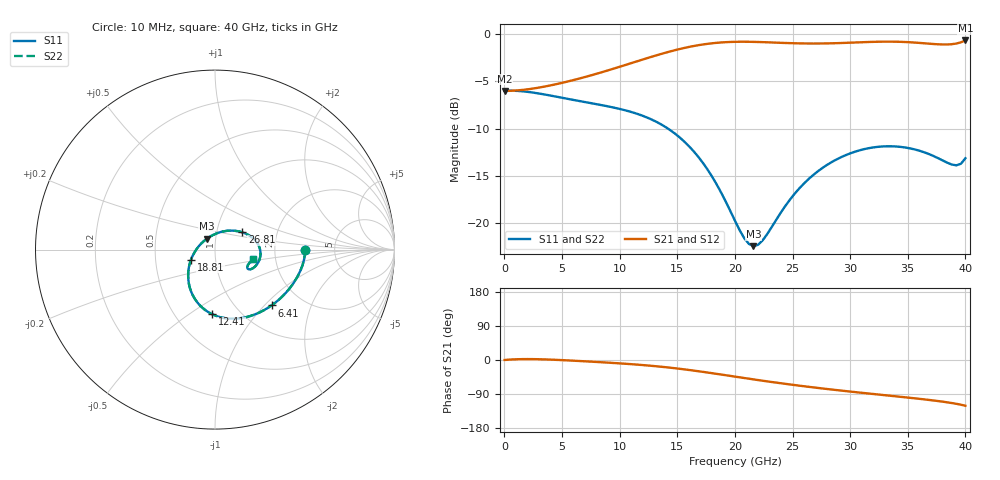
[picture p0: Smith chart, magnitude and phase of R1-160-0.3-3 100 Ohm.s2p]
!version-1
!date-09.2020
# MHz S RI R 50
!Freq ReS11 ImS11 ReS21 ImS21 ReS12 ImS12 ReS22 ImS22
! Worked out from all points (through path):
!   101 points, 10 MHz to 40 GHz, reference 50 ohm
!   highest |S21| = -0.70 dB at 40 GHz (marker M1); lowest = -6.0 dB at 10 MHz (marker M2)
!   group delay of S21, straight-line fit = 9.25 ps
!   lowest |S11| = -22.4 dB at 21.61 GHz (marker M3), VSWR 1.16, Z = 45.3 + j5.51 ohm
!   |S11| at or under -10 dB: 14.18 GHz to end of sweep
!   |S22| runs from -22.4 to -6.0 dB; largest |S21 - S12| = 0
!   S11 on the Smith chart (normalised r, x): 10 MHz: 3.00, -0.00; 6.41 GHz: 1.42, -1.10; 12.41 GHz: 0.75, -0.62; 18.81 GHz: 0.76, -0.09; 26.81 GHz: 1.33, +0.26; 40 GHz: 1.53, -0.18
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10  0.5 -0.000398  0.5 0.000242  0.5 0.000242  0.5 -0.000398
2810  0.466 -0.1382  0.5176 0.0194  0.5176 0.0194  0.466 -0.1382
6410  0.3153 -0.3111  0.5782 -0.0255  0.5782 -0.0255  0.3153 -0.3111
6810  0.2939 -0.3252  0.5866 -0.0326  0.5866 -0.0326  0.2939 -0.3252
9610  0.1361 -0.383  0.652 -0.0933  0.652 -0.0933  0.1361 -0.383
12410  -0.0149 -0.3606  0.7213 -0.1855  0.7213 -0.1855  -0.0149 -0.3606
13610  -0.0691 -0.325  0.7455 -0.24  0.7455 -0.24  -0.0691 -0.325
16410  -0.1452 -0.1914  0.7613 -0.4034  0.7613 -0.4034  -0.1452 -0.1914
17610  -0.1487 -0.1227  0.7421 -0.4821  0.7421 -0.4821  -0.1487 -0.1227
18810  -0.1337 -0.0562  0.7054 -0.5589  0.7054 -0.5589  -0.1337 -0.0562
20010  -0.103 0.00218  0.6536 -0.6287  0.6536 -0.6287  -0.103 0.00218
20810  -0.076 0.0344  0.6128 -0.6697  0.6128 -0.6697  -0.076 0.0344
21610  -0.0457 0.0604  0.5686 -0.7058  0.5686 -0.7058  -0.0457 0.0604
22410  -0.0135 0.0803  0.5224 -0.7371  0.5224 -0.7371  -0.0135 0.0803
24810  0.0829 0.1056  0.3818 -0.8067  0.3818 -0.8067  0.0829 0.1056
26810  0.1524 0.0962  0.2702 -0.8464  0.2702 -0.8464  0.1524 0.0962
30010  0.2298 0.0446  0.1042 -0.8915  0.1042 -0.8915  0.2298 0.0446
33610  0.2514 -0.0423  -0.0752 -0.9057  -0.0752 -0.9057  0.2514 -0.0423
35610  0.2289 -0.0884  -0.174 -0.8818  -0.174 -0.8818  0.2289 -0.0884
37610  0.1915 -0.1104  -0.2762 -0.8357  -0.2762 -0.8357  0.1915 -0.1104
39210  0.1826 -0.0872  -0.3836 -0.8009  -0.3836 -0.8009  0.1826 -0.0872
40000  0.2135 -0.055  -0.4711 -0.7927  -0.4711 -0.7927  0.2135 -0.055
